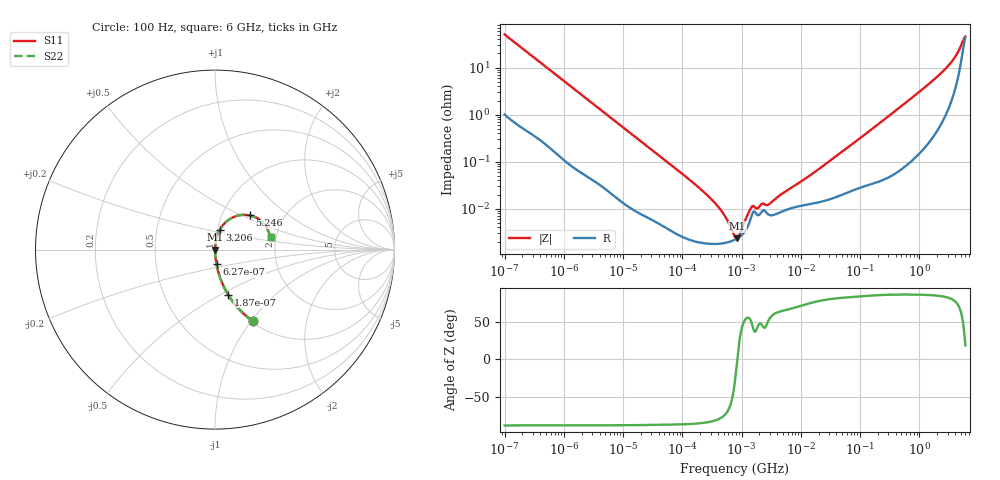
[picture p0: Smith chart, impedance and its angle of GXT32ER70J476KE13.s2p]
!Murata Part Number: GXT32ER70J476KE13
!These Parameters are Measured in Series Mode Connection
!Data Generated on Jan 08, 2026
!  o--ll--o
!Port1  Port2
!  o------o
!Operation Temp=25[degC], DC Bias Voltage=0[V]
!Freq. Start=100[Hz] Stop=6[GHz] 401[Steps]
# Hz S RI R 50
!Freq.(Hz) S11(Real) S11(Imag) S21(Real) S21(Imag) S12(Real) S12(Imag) S22(Real) S22(Imag)
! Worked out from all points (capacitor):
!   401 points, 100 Hz to 6 GHz, reference 50 ohm
!   read as one part in series: C = 31.3 uF near 109 Hz
!   lowest |Z| = 2.35 mohm at 847.2 kHz (marker M1)
!   series resonance near 845.4 kHz, so ESL is about 1.1 nH
!   S11 on the Smith chart (normalised r, x): 100 Hz: 1.02, -1.01; 187 Hz: 1.01, -0.54; 627 Hz: 1.00, -0.17; 3.206 GHz: 1.03, +0.23; 5.246 GHz: 1.35, +0.56; 6 GHz: 1.87, +0.30
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100  0.2091 -0.3968  0.7909 0.3968  0.7909 0.3968  0.2091 -0.3968
187  0.0734 -0.251  0.9266 0.251  0.9266 0.251  0.0734 -0.251
320  0.0283 -0.1552  0.9717 0.1552  0.9717 0.1552  0.0283 -0.1552
627  0.00856 -0.0819  0.9914 0.0819  0.9914 0.0819  0.00856 -0.0819
2008  0.00125 -0.0261  0.9987 0.0261  0.9987 0.0261  0.00125 -0.0261
40335  4.98e-05 -0.00136  1 0.00136  1 0.00136  4.98e-05 -0.00136
184852  1.95e-05 -0.00029  1 0.00029  1 0.00029  1.95e-05 -0.00029
413847  1.8e-05 -0.000105  1 0.000105  1 0.000105  1.8e-05 -0.000105
473344  1.84e-05 -8.27e-05  1 8.27e-05  1 8.27e-05  1.84e-05 -8.27e-05
774597  2.21e-05 -1.21e-05  1 1.21e-05  1 1.21e-05  2.21e-05 -1.21e-05
847162  2.35e-05 3e-07  1 -3e-07  1 -3e-07  2.35e-05 3e-07
1813585  7.53e-05 6.65e-05  0.9999 -6.65e-05  0.9999 -6.65e-05  7.53e-05 6.65e-05
2268635  9.16e-05 9.14e-05  0.9999 -9.14e-05  0.9999 -9.14e-05  9.16e-05 9.14e-05
2837864  7.53e-05 9.68e-05  0.9999 -9.68e-05  0.9999 -9.68e-05  7.53e-05 9.68e-05
4643984  8.54e-05 0.000182  0.9999 -0.000182  0.9999 -0.000182  8.54e-05 0.000182
1.555665e7  0.000129 0.000537  0.9999 -0.000537  0.9999 -0.000537  0.000129 0.000537
3.124326e8  0.000565 0.00957  0.9994 -0.00957  0.9994 -0.00957  0.000565 0.00957
1.497423e9  0.0048 0.0461  0.9952 -0.0461  0.9952 -0.0461  0.0048 0.0461
3.205649e9  0.027 0.1103  0.973 -0.1103  0.973 -0.1103  0.027 0.1103
4.385646e9  0.0818 0.1699  0.9182 -0.1699  0.9182 -0.1699  0.0818 0.1699
5.245841e9  0.1929 0.1919  0.8071 -0.1919  0.8071 -0.1919  0.1929 0.1919
6e9  0.3099 0.0714  0.6901 -0.0714  0.6901 -0.0714  0.3099 0.0714
